FUNCTION "CARICO_SCAR_PRESSA" : VOID
TITLE =BLOCK CLUTCH/BRAKE
AUTHOR : Esposito
FAMILY : EGAL_srl
NAME : CLUTCH
VERSION : 0.1

BEGIN
NETWORK
TITLE =CONDITIONS FOR ENABLE CLUTCH/BRAKE WITH OVERLOAD
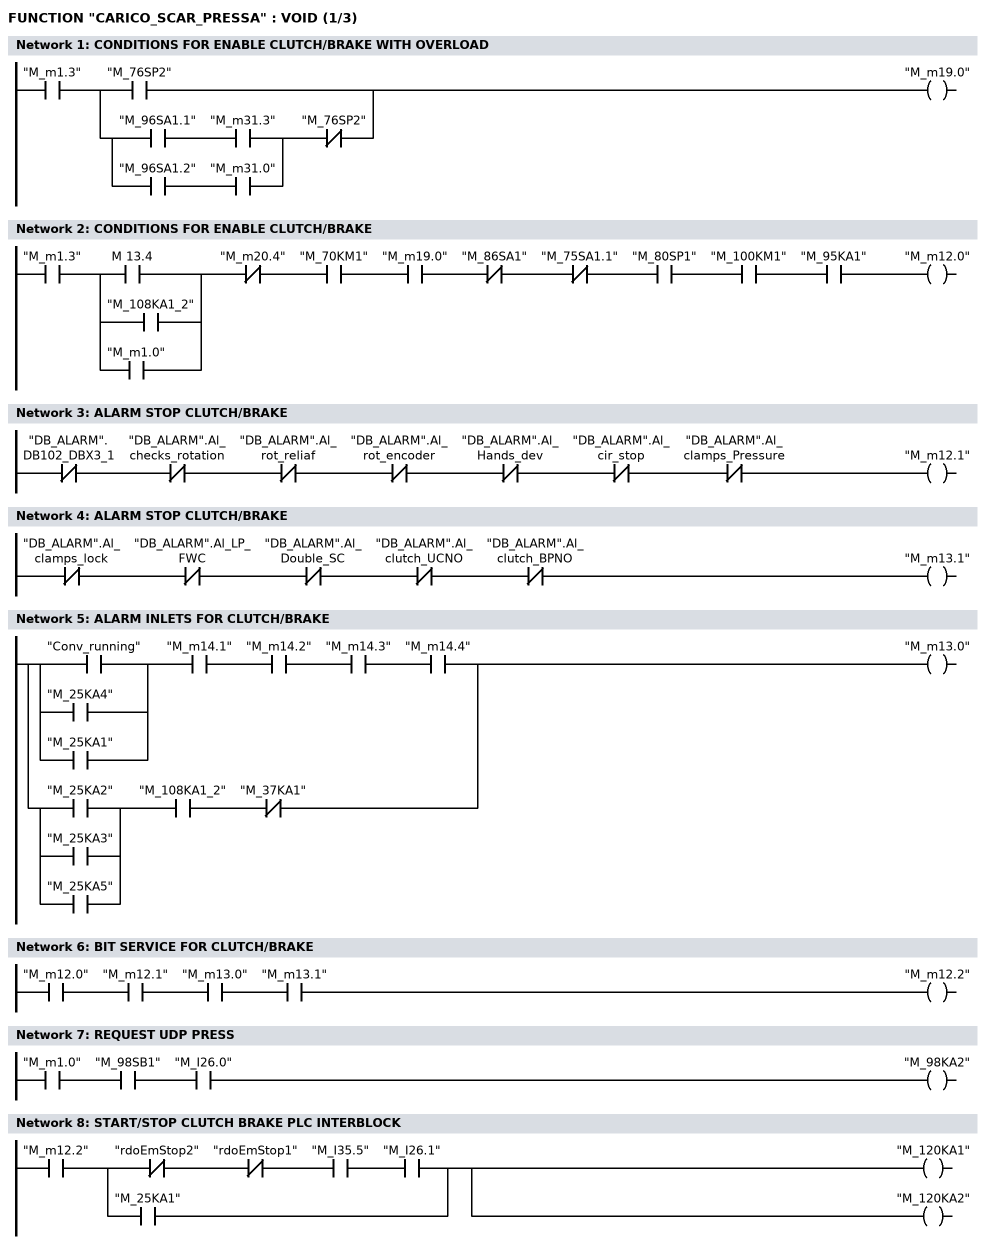
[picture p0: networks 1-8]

      U     "M_m1.3";
      U(    ;
      O     "M_76SP2";
      O     ;
      U(    ;
      U     "M_96SA1.1";
      U     "M_m31.3";
      O     ;
      U     "M_96SA1.2";
      U     "M_m31.0";
      )     ;
      UN    "M_76SP2";
      )     ;
      =     "M_m19.0";
NETWORK
TITLE =CONDITIONS FOR ENABLE CLUTCH/BRAKE

      U     "M_m1.3";
      U(    ;
      O     M     13.4;
      O     "M_108KA1_2";
      O     "M_m1.0";
      )     ;
      UN    "M_m20.4";
      U     "M_70KM1";
      U     "M_m19.0";
      UN    "M_86SA1";
      UN    "M_75SA1.1";
      U     "M_80SP1";
      U     "M_100KM1";
      U     "M_95KA1";
      =     "M_m12.0";
NETWORK
TITLE =ALARM STOP CLUTCH/BRAKE

      UN    "DB_ALARM".DB102_DBX3_1;
      UN    "DB_ALARM".Al_checks_rotation;
      UN    "DB_ALARM".Al_rot_reliaf;
      UN    "DB_ALARM".Al_rot_encoder;
      UN    "DB_ALARM".Al_Hands_dev;
      UN    "DB_ALARM".Al_cir_stop;
      UN    "DB_ALARM".Al_clamps_Pressure;
      =     "M_m12.1";
NETWORK
TITLE =ALARM STOP CLUTCH/BRAKE

      UN    "DB_ALARM".Al_clamps_lock;
      UN    "DB_ALARM".Al_LP_FWC;
      UN    "DB_ALARM".Al_Double_SC;
      UN    "DB_ALARM".Al_clutch_UCNO;
      UN    "DB_ALARM".Al_clutch_BPNO;
      =     "M_m13.1";
NETWORK
TITLE =ALARM INLETS FOR CLUTCH/BRAKE

      U(    ;
      O     "Conv_running";
      O     "M_25KA4";
      O     "M_25KA1";
      )     ;
      U     "M_m14.1";
      U     "M_m14.2";
      U     "M_m14.3";
      U     "M_m14.4";
      O     ;
      U(    ;
      O     "M_25KA2";
      O     "M_25KA3";
      O     "M_25KA5";
      )     ;
      U     "M_108KA1_2";
      UN    "M_37KA1";
      =     "M_m13.0";
NETWORK
TITLE =BIT SERVICE FOR CLUTCH/BRAKE

      U     "M_m12.0";
      U     "M_m12.1";
      U     "M_m13.0";
      U     "M_m13.1";
      =     "M_m12.2";
NETWORK
TITLE =REQUEST UDP PRESS

      U     "M_m1.0";
      U     "M_98SB1";
      U     "M_I26.0";
      =     "M_98KA2";
NETWORK
TITLE =START/STOP CLUTCH BRAKE PLC INTERBLOCK

      U     "M_m12.2";
      U(    ;
      UN    "rdoEmStop2";
      UN    "rdoEmStop1";
      U     "M_I35.5";
      U     "M_I26.1";
      O     "M_25KA1";
      )     ;
      =     "M_120KA1";
      =     "M_120KA2";
NETWORK
TITLE =RESET FLIP/FLOP M16.0
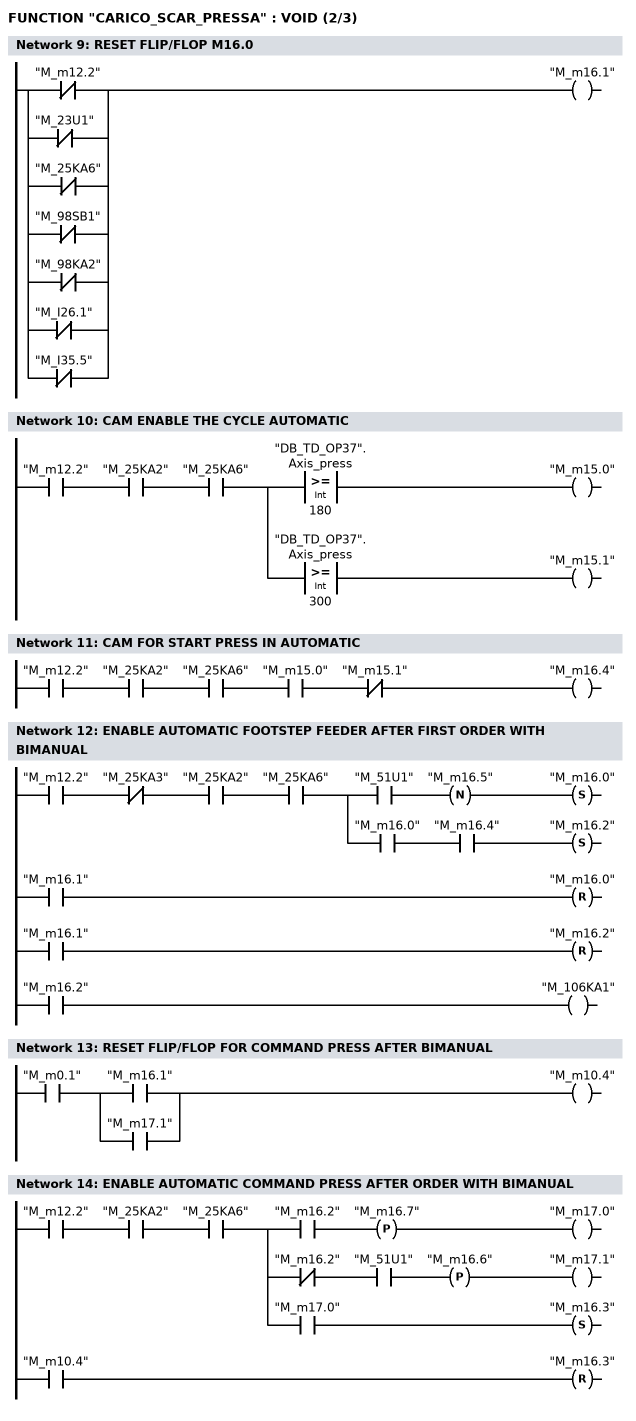
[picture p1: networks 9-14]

      ON    "M_m12.2";
      ON    "M_23U1";
      ON    "M_25KA6";
      ON    "M_98SB1";
      ON    "M_98KA2";
      ON    "M_I26.1";
      ON    "M_I35.5";
      =     "M_m16.1";
NETWORK
TITLE =CAM ENABLE THE CYCLE AUTOMATIC

      U     "M_m12.2";
      U     "M_25KA2";
      U     "M_25KA6";
      =     L      0.0;
      U     L      0.0;
      U(    ;
      L     "DB_TD_OP37".Axis_press;
      L     180;
      >=I   ;
      )     ;
      =     "M_m15.0";
      U     L      0.0;
      U(    ;
      L     "DB_TD_OP37".Axis_press;
      L     300;
      >=I   ;
      )     ;
      =     "M_m15.1";

NETWORK
TITLE =CAM FOR START PRESS IN AUTOMATIC

      U     "M_m12.2";
      U     "M_25KA2";
      U     "M_25KA6";
      U     "M_m15.0";
      UN    "M_m15.1";
      =     "M_m16.4";
NETWORK
TITLE =ENABLE AUTOMATIC FOOTSTEP FEEDER AFTER FIRST ORDER WITH BIMANUAL

      U     "M_m12.2";
      UN    "M_25KA3";
      U     "M_25KA2";
      U     "M_25KA6";
      =     L      0.0;
      U     L      0.0;
      U     "M_51U1";
      FN    "M_m16.5";
      S     "M_m16.0";
      U     "M_m16.1";
      R     "M_m16.0";
      NOP   0;
      U     L      0.0;
      U     "M_m16.0";
      U     "M_m16.4";
      S     "M_m16.2";
      U     "M_m16.1";
      R     "M_m16.2";
      U     "M_m16.2";
      =     "M_106KA1";
NETWORK
TITLE =RESET FLIP/FLOP FOR COMMAND PRESS AFTER BIMANUAL

      U     "M_m0.1";
      U(    ;
      O     "M_m16.1";
      O     "M_m17.1";
      )     ;
      =     "M_m10.4";
NETWORK
TITLE =ENABLE AUTOMATIC COMMAND PRESS AFTER ORDER WITH BIMANUAL

      U     "M_m12.2";
      U     "M_25KA2";
      U     "M_25KA6";
      =     L      0.0;
      U     L      0.0;
      U     "M_m16.2";
      FP    "M_m16.7";
      =     "M_m17.0";
      U     L      0.0;
      UN    "M_m16.2";
      U     "M_51U1";
      FP    "M_m16.6";
      =     "M_m17.1";
      U     L      0.0;
      U     "M_m17.0";
      S     "M_m16.3";
      U     "M_m10.4";
      R     "M_m16.3";
      NOP   0;
NETWORK
TITLE =RESET FLIP/FLOP ROBOT IN AUTOMATIC
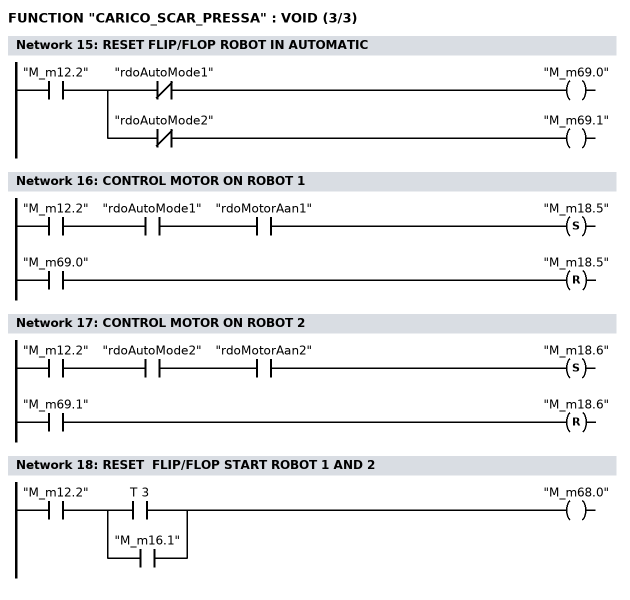
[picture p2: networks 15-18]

      U     "M_m12.2";
      =     L      0.0;
      U     L      0.0;
      UN    "rdoAutoMode1";
      =     "M_m69.0";
      U     L      0.0;
      UN    "rdoAutoMode2";
      =     "M_m69.1";
NETWORK
TITLE =CONTROL MOTOR ON ROBOT 1

      U     "M_m12.2";
      U     "rdoAutoMode1";
      U     "rdoMotorAan1";
      S     "M_m18.5";
      U     "M_m69.0";
      R     "M_m18.5";
      NOP   0;
NETWORK
TITLE =CONTROL MOTOR ON ROBOT 2

      U     "M_m12.2";
      U     "rdoAutoMode2";
      U     "rdoMotorAan2";
      S     "M_m18.6";
      U     "M_m69.1";
      R     "M_m18.6";
      NOP   0;
NETWORK
TITLE =RESET  FLIP/FLOP START ROBOT 1 AND 2

      U     "M_m12.2";
      U(    ;
      O     T      3;
      O     "M_m16.1";
      )     ;
      =     "M_m68.0";
NETWORK
TITLE =CONTROL ROBOT AL FIRST START

      U     "M_m12.2";
      =     L      0.0;
      U     L      0.0;
      U     "M_m16.3";
      U(    ;
      O     "rdoAutoMode1";
      O     "rdoAutoMode2";
      )     ;
      S     M     28.0;
      U     M     28.1;
      R     M     28.0;
      NOP   0;
      U     L      0.0;
      U     "M_I35.0";
      L     S5T#3S;
      SS    T     66;
      U     L      0.0;
      U     T     66;
      =     M     28.1;
NETWORK
TITLE =START FROM ROBOT 1 IN CYCLE  0 AND 1
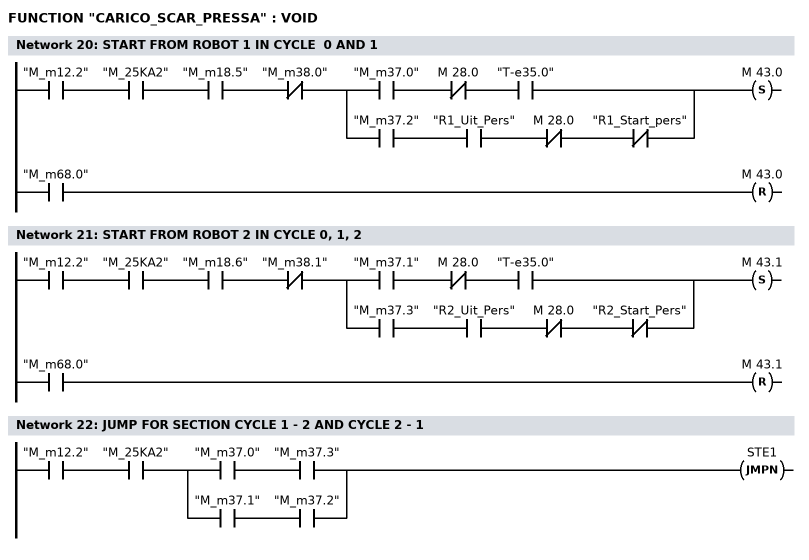
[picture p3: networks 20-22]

      U     "M_m12.2";
      U     "M_25KA2";
      U     "M_m18.5";
      UN    "M_m38.0";
      U(    ;
      U     "M_m37.0";
      UN    M     28.0;
      U     "T-e35.0";
      O     ;
      U     "M_m37.2";
      U     "R1_Uit_Pers";
      UN    M     28.0;
      UN    "R1_Start_pers";
      )     ;
      S     M     43.0;
      U     "M_m68.0";
      R     M     43.0;
      NOP   0;
NETWORK
TITLE =START FROM ROBOT 2 IN CYCLE 0, 1, 2

      U     "M_m12.2";
      U     "M_25KA2";
      U     "M_m18.6";
      UN    "M_m38.1";
      U(    ;
      U     "M_m37.1";
      UN    M     28.0;
      U     "T-e35.0";
      O     ;
      U     "M_m37.3";
      U     "R2_Uit_Pers";
      UN    M     28.0;
      UN    "R2_Start_Pers";
      )     ;
      S     M     43.1;
      U     "M_m68.0";
      R     M     43.1;
      NOP   0;
NETWORK
TITLE =JUMP FOR SECTION CYCLE 1 - 2 AND CYCLE 2 - 1

      U     "M_m12.2";
      U     "M_25KA2";
      U(    ;
      U     "M_m37.0";
      U     "M_m37.3";
      O     ;
      U     "M_m37.1";
      U     "M_m37.2";
      )     ;
      SPBN  STE1;
NETWORK
TITLE =CONTROL FOGLIO IN PRESS AND CENTERTABLE IN CYCLE 1 - 2

      U     "M_m12.2";
      =     L      0.0;
      U     L      0.0;
      U(    ;
      O     "M_115SQ1";
      O     ;
      U     "m-M36.5";
      U     "M_I35.0";
      )     ;
      S     "m-M18.4";
      U     M     18.7;
      R     "m-M18.4";
      NOP   0;
      U     L      0.0;
      UN    "R1_In_Pers";
      UN    "R2_In_Pers";
      UN    "M_115SQ1";
      U(    ;
      U     "m-M36.5";
      U     "T-e35.0";
      O     ;
      U     "m-M36.6";
      U     "M_I35.0";
      )     ;
      UN    M     33.1;
      =     L      0.1;
      U     L      0.1;
      BLD   102;
      L     S5T#50MS;
      SI    T     15;
      U     L      0.1;
      U     T     15;
      =     M     18.7;
NETWORK
TITLE =SELEZIONE START PASSO FEEDER
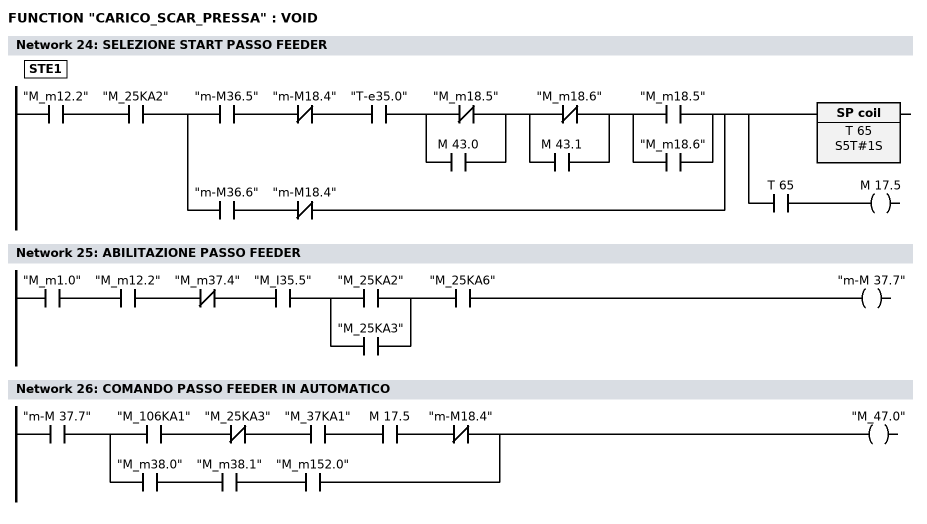
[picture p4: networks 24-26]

STE1: U     "M_m12.2";
      U     "M_25KA2";
      U(    ;
      U     "m-M36.5";
      UN    "m-M18.4";
      U     "T-e35.0";
//      UN    M     91.1
      U(    ;
      ON    "M_m18.5";
      O     M     43.0;
      )     ;
      U(    ;
      ON    "M_m18.6";
      O     M     43.1;
      )     ;
      U(    ;
      O     "M_m18.5";
      O     "M_m18.6";
      )     ;
      O     ;
      U     "m-M36.6";
      UN    "m-M18.4";
      )     ;
      =     L      0.0;
      U     L      0.0;
      BLD   102;
      L     S5T#1S;
      SI    T     65;
      U     L      0.0;
      U     T     65;
      =     M     17.5;
NETWORK
TITLE =ABILITAZIONE PASSO FEEDER

      U     "M_m1.0";
      U     "M_m12.2";
      UN    "M_m37.4";
      U     "M_I35.5";
      U(    ;
      O     "M_25KA2";
      O     "M_25KA3";
      )     ;
      U     "M_25KA6";
      =     "m-M 37.7";


NETWORK
TITLE =COMANDO PASSO FEEDER IN AUTOMATICO

      U     "m-M 37.7";
      U(    ;
      U     "M_106KA1";
      UN    "M_25KA3";
      U     "M_37KA1";
      U     M     17.5;
      UN    "m-M18.4";
      O     ;
      U     "M_m38.0";
      U     "M_m38.1";
      U     "M_m152.0";
      )     ;
      =     "M_47.0";
NETWORK
TITLE =CONTROL BLANKCART IN PRESS > CENTERTABLE

      U     "M_m1.0";
      =     L      0.0;
      U     L      0.0;
      U     "M_115SQ1";
      S     M     33.1;
      U     M     33.4;
      R     M     33.1;
      NOP   0;
      U     L      0.0;
      U(    ;
      O     "M_I35.0";
      ON    "M_25KA6";
      )     ;
      =     M     33.4;
NETWORK
TITLE =CONTROL BLANKCART IN CENTERTABLE FOR RESET FEEDER

      U     "M_m12.2";
      U     "M_25KA2";
      U     "M_I35.0";
      =     L      0.0;
      U     L      0.0;
      FP    M     91.0;
      S     M     91.1;
      U     M     91.3;
      R     M     91.1;
      NOP   0;
      U     L      0.0;
      FN    M     91.2;
      =     M     91.3;
NETWORK
TITLE =RESET FLIP/FLOP START FEEDER
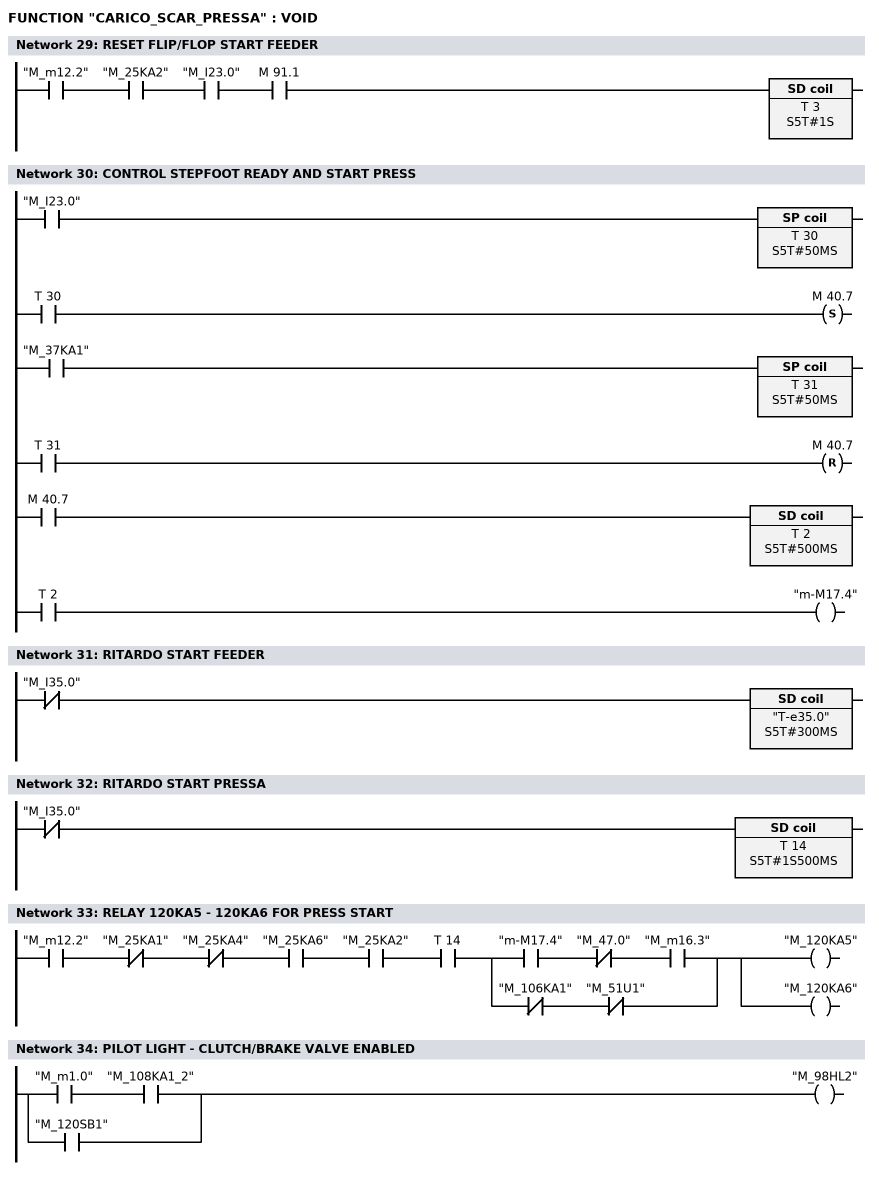
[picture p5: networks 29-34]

      U     "M_m12.2";
      U     "M_25KA2";
      U     "M_I23.0";
      U     M     91.1;
      L     S5T#1S;
      SE    T      3;
NETWORK
TITLE =CONTROL STEPFOOT READY AND START PRESS


      U     "M_I23.0";
      L     S5T#50MS;
      SI    T     30;

      U     T     30;
      S     M     40.7;

      U     "M_37KA1";
      L     S5T#50MS;
      SI    T     31;

      U     T     31;
      R     M     40.7;

      U     M     40.7;
      L     S5T#500MS;
      SE    T      2;

      U     T      2;
      =     "m-M17.4";
NETWORK
TITLE =RITARDO START FEEDER

      UN    "M_I35.0";
      L     S5T#300MS;
      SE    "T-e35.0";


NETWORK
TITLE =RITARDO START PRESSA

      UN    "M_I35.0";
      L     S5T#1S500MS;
      SE    T     14;


NETWORK
TITLE =RELAY 120KA5 - 120KA6 FOR PRESS START

      U     "M_m12.2";
      UN    "M_25KA1";
      UN    "M_25KA4";
      U     "M_25KA6";
      U     "M_25KA2";
      U     T     14;
      U(    ;
      U     "m-M17.4";
      UN    "M_47.0";
      U     "M_m16.3";
      O     ;
      UN    "M_106KA1";
      UN    "M_51U1";
      )     ;
      =     "M_120KA5";
      =     "M_120KA6";
NETWORK
TITLE =PILOT LIGHT - CLUTCH/BRAKE VALVE ENABLED

      U     "M_m1.0";
      U     "M_108KA1_2";
      O     "M_120SB1";
      =     "M_98HL2";
END_FUNCTION

